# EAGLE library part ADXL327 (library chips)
ADXL327 3-Axis Analog Accelerometer
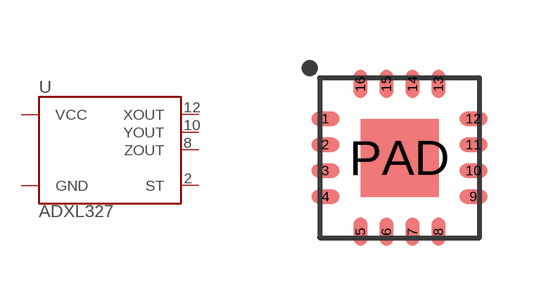
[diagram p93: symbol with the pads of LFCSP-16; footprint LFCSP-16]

Designator prefix U

## ADXL327 (DIGIKEY: ADXL327BCPZ-ND)  [LFCSP-16]
2  ST
3  GND
5  GND
6  GND
7  GND
8  ZOUT
10  YOUT
12  XOUT
14  VCC
15  VCC

## Footprint LFCSP-16 (pad centres in mm)
smd 0.7 x 0.35: 1 -1.85,0.975; 2 -1.85,0.325; 3 -1.85,-0.325; 4 -1.85,-0.975; 9 1.85,-0.975; 10 1.85,-0.325; 11 1.85,0.325; 12 1.85,0.975
smd 0.35 x 0.7: 5 -0.975,-1.85; 6 -0.325,-1.85; 7 0.325,-1.85; 8 0.975,-1.85; 13 0.975,1.85; 14 0.325,1.85; 15 -0.325,1.85; 16 -0.975,1.85
smd 1.95 x 1.95: PAD 0,0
